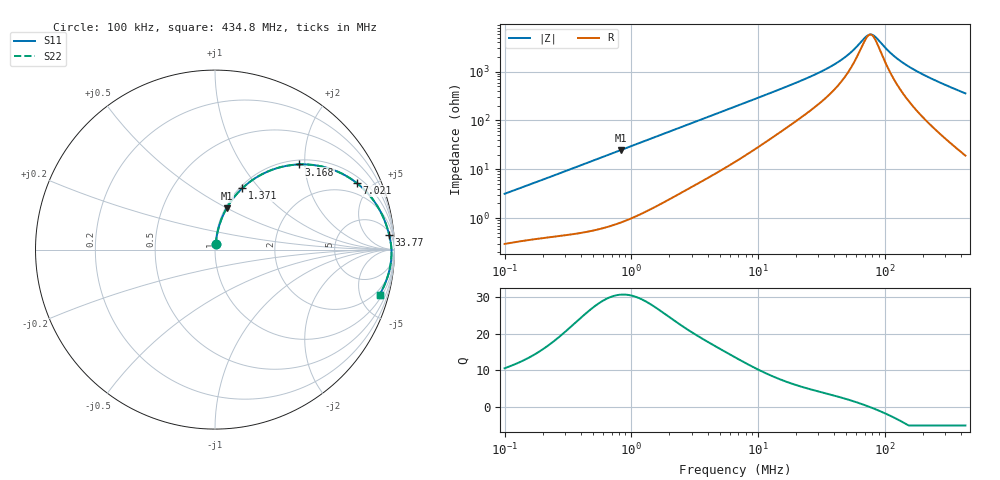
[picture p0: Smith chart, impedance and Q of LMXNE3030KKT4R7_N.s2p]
! LMXNE3030KKT4R7_N  S-PARAMETER MODEL  ( General Type )
! Model Generated by TAIYO YUDEN Corporation (https://www.yuden.co.jp/en/)
! Version 1.0
! TAIYO YUDEN Control No. 191023NI43SB-FBB
! Copyright(c) 2019 TAIYO YUDEN CO.,LTD. All Rights Reserved.
! Product Description (link to TY-COMPAS)
! https://ds.yuden.co.jp/TYCOMPAS/or/detail?pn=LMXNE3030KKT4R7MN&u=M
! Products Name : Inductors
! Characteristics :
!  Inductance : 4.7 uH , SRF(min) : 50 MHz , DC Resistance(max) : 0.204 Ohm
!  Rated Current : Saturation :850 mA , Temp Rise : 900 mA (40 degC)
!  Case Size : 3.0 x 3.0 / 0.118 x 0.118 [mm/inch] , Thickness : 1 / 0.039 [mm/inch]
!  (Conditions: Temperature = 25 degC , DC Bias Current/Voltage = 0A / 0V)
! External Node Assignments :
!  1  o---GGG---o  2
! GND o---------o GND
! Frequency Range : 0.1MHz  -  434.768421MHz  [ 402 STEP ]
# MHz S RI R 50
! Freq[MHz].  S11 Real  S11 Imag  S21 Real  S21 Imag  S12 Real  S12 Imag  S22 Real  S22 Imag
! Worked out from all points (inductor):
!   401 points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, 100 kHz to 434.8 MHz, reference 50 ohm
!   read as one part in series: L = 4.92 uH near 104.3 kHz
!   highest Q = 30.7 at 829.2 kHz (marker M1), where L = 4.77 uH
!   self-resonance near 76.99 MHz
!   S11 on the Smith chart (normalised r, x): 100 kHz: 1.01, +0.06; 1.371 MHz: 1.03, +0.82; 3.168 MHz: 1.09, +1.87; 7.021 MHz: 1.31, +4.08; 33.77 MHz: 7, +21; 434.8 MHz: 1.38, -7.18
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0.1  0.0039 0.031  0.9961 -0.031  0.9961 -0.031  0.0039 0.031
0.406826  0.0195 0.1196  0.9805 -0.1196  0.9805 -0.1196  0.0195 0.1196
0.829202  0.0648 0.2305  0.9352 -0.2305  0.9352 -0.2305  0.0648 0.2305
1.370742  0.152 0.3419  0.848 -0.3419  0.848 -0.3419  0.152 0.3419
1.65507  0.2043 0.3848  0.7957 -0.3848  0.7957 -0.3848  0.2043 0.3848
3.167973  0.4675 0.4745  0.5325 -0.4745  0.5325 -0.4745  0.4675 0.4745
4.429062  0.6208 0.4566  0.3792 -0.4566  0.3792 -0.4566  0.6208 0.4566
6.733248  0.7775 0.3804  0.2225 -0.3804  0.2225 -0.3804  0.7775 0.3804
7.021274  0.79 0.3709  0.21 -0.3709  0.21 -0.3709  0.79 0.3709
12.35943  0.905 0.2417  0.095 -0.2417  0.095 -0.2417  0.905 0.2417
26.82484  0.9627 0.1114  0.0373 -0.1114  0.0373 -0.1114  0.9627 0.1114
33.77453  0.9703 0.0834  0.0297 -0.0834  0.0297 -0.0834  0.9703 0.0834
49.23919  0.9786 0.0433  0.0214 -0.0433  0.0214 -0.0433  0.9786 0.0433
57.01386  0.9806 0.0289  0.0194 -0.0289  0.0194 -0.0289  0.9806 0.0289
70.29701  0.9826 0.00873  0.0174 -0.00873  0.0174 -0.00873  0.9826 0.00873
76.43979  0.983 0.000691  0.017 -0.000691  0.017 -0.000691  0.983 0.000691
84.8785  0.9834 -0.00944  0.0166 0.00944  0.0166 0.00944  0.9834 -0.00944
109.1303  0.9831 -0.0346  0.0169 0.0346  0.0169 0.0346  0.9831 -0.0346
137.4034  0.9811 -0.0597  0.0189 0.0597  0.0189 0.0597  0.9811 -0.0597
184.2199  0.9757 -0.096  0.0243 0.096  0.0243 0.096  0.9757 -0.096
280.0589  0.9584 -0.161  0.0416 0.161  0.0416 0.161  0.9584 -0.161
434.7684  0.9169 -0.2508  0.0831 0.2508  0.0831 0.2508  0.9169 -0.2508
